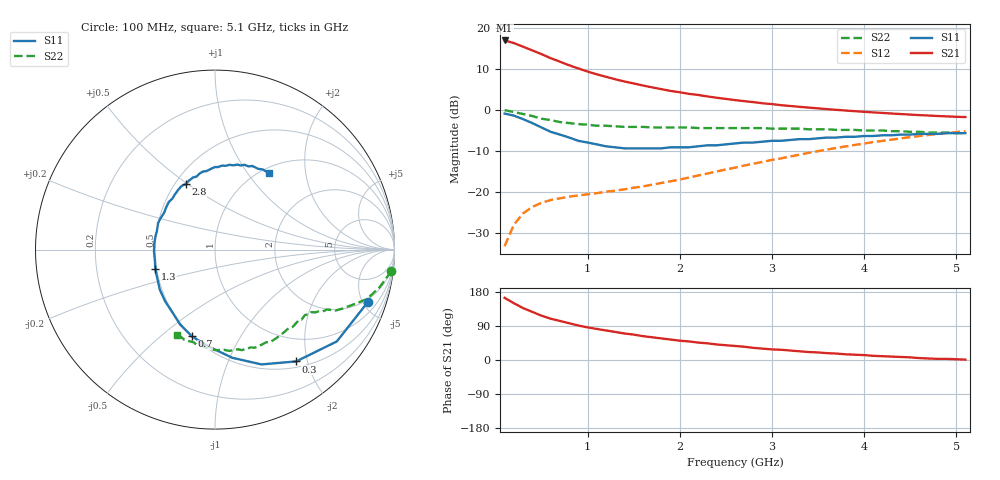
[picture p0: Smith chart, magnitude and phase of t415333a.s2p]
!AT-41533
!S and NOISE PARAMETERS at Vce=2.7V Ic=2mA. LAST UPDATED 01-25-95
# ghz s ma r 50
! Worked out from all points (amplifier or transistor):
!   51 points, 100 MHz to 5.1 GHz, reference 50 ohm
!   highest |S21| = 16.9 dB at 100 MHz (marker M1)
!   |S21| within 3 dB of that: start of sweep to 464.7 MHz
!   unconditionally stable (mu >= 1): 1.247 GHz to 2.505 GHz
!   at 900 MHz: K = 0.81, MSG = 15.4 dB, |S12| = -20.8 dB
!   at 2.6 GHz: K = 0.98, MSG = 8.2 dB, |S12| = -14.1 dB
!   at 5.1 GHz: K = 0.85, MSG = 1.7 dB, |S12| = -5.2 dB
!   lowest NFmin = 0.70 dB at 100 MHz
!   S11 on the Smith chart (normalised r, x): 100 MHz: 1.76, -5.42; 300 MHz: 0.59, -1.81; 700 MHz: 0.50, -0.64; 1.3 GHz: 0.49, -0.12; 2.8 GHz: 0.57, +0.49; 5.1 GHz: 1.08, +1.26
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0.1  0.9 -19.0  6.966 164.0  0.022 79.0  0.99 -7.0
0.2  0.85 -37.0  6.478 150.0  0.04 70.0  0.94 -13.0
0.3  0.77 -54.0  5.85 137.0  0.055 62.0  0.89 -18.0
0.4  0.69 -68.0  5.281 127.0  0.066 57.0  0.84 -21.0
0.5  0.61 -81.0  4.751 117.0  0.074 52.0  0.78 -25.0
0.6  0.54 -94.0  4.243 109.0  0.08 49.0  0.75 -27.0
0.7  0.5 -105.0  3.847 103.0  0.084 48.0  0.71 -28.0
0.8  0.46 -115.0  3.48 97.0  0.088 47.0  0.69 -30.0
0.9  0.42 -125.0  3.184 91.0  0.091 47.0  0.67 -31.0
1  0.4 -134.0  2.913 86.0  0.094 47.0  0.66 -32.0
1.1  0.38 -144.0  2.701 82.0  0.097 49.0  0.64 -33.0
1.3  0.35 -162.0  2.352 74.0  0.104 51.0  0.63 -35.0
1.4  0.34 -170.0  2.209 70.0  0.108 52.0  0.62 -36.0
1.6  0.34 175.0  1.975 63.0  0.117 56.0  0.62 -39.0
1.8  0.34 162.0  1.784 57.0  0.129 58.0  0.61 -41.0
2  0.35 150.0  1.635 51.0  0.142 61.0  0.61 -44.0
2.2  0.36 139.0  1.516 46.0  0.159 63.0  0.6 -47.0
2.6  0.39 122.0  1.313 37.0  0.198 64.0  0.6 -53.0
2.8  0.4 114.0  1.24 32.0  0.221 64.0  0.6 -57.0
3.5  0.45 93.0  1.041 20.0  0.314 60.0  0.58 -73.0
4.3  0.49 73.0  0.901 9.0  0.434 49.0  0.55 -93.0
5.1  0.52 55.0  0.816 1.0  0.55 37.0  0.52 -114.0
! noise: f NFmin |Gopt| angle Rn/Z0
0.1  0.7  0.58  7  0.28
0.9  1  0.44  86  0.17
1.8  1.5  0.47  -172  0.06
2.4  1.9  0.62  -132  0.15
